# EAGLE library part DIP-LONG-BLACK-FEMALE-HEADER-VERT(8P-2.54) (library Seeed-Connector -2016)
320030013
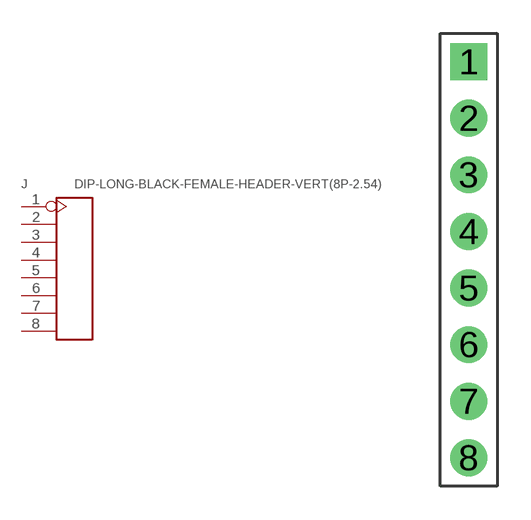
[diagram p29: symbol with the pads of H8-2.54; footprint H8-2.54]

Designator prefix J

## DIP-LONG-BLACK-FEMALE-HEADER-VERT(8P-2.54) (MPN: F185-2108A1BSYA1; VALUE: 8p-2.54)  [H8-2.54]
1  1
2  2
3  3
4  4
5  5
6  6
7  7
8  8

## Footprint H8-2.54 (pad centres in mm)
drill 0.889 pad 1.651 square: 1 0,8.89
drill 0.889 pad 1.651: 2 0,6.35; 3 0,3.81; 4 0,1.27; 5 0,-1.27; 6 0,-3.81; 7 0,-6.35; 8 0,-8.89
